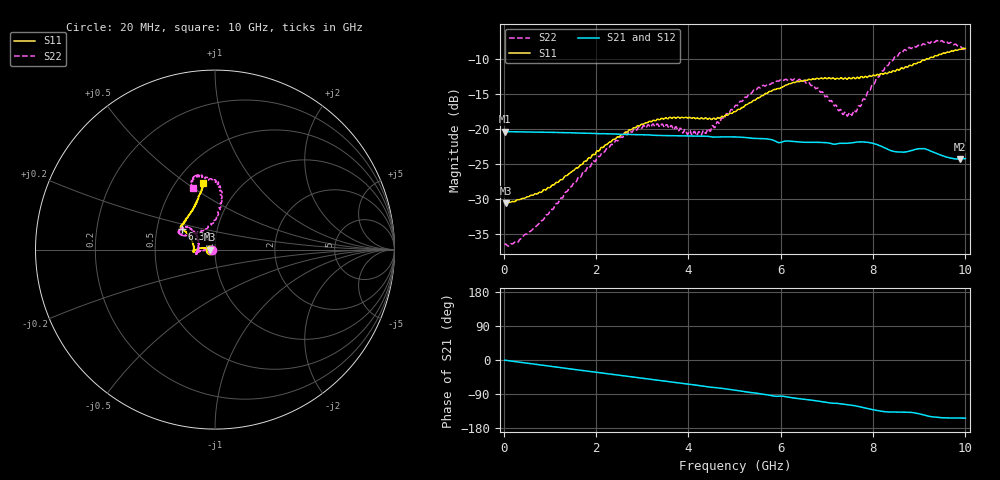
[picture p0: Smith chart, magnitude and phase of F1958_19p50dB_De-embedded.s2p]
! Integrated Device Technology
! Corporate Headquarters
! 6024 Silver Creek Valley Road
! San Jose, CA 95138  USA
! Phone:  1-408-284-8200
! Toll Free:  1-800-223-1366
! Webpage:  http://www.idt.com/
! Timing and RF Division
! 515 Groton Road, Suite 102
! Westford, MA 01886-6024
! Device:  F1958
! Description: 7-bit 0.25 dB Digital Step Attenuator
! Frequency:  0.001 -  6.000 GHz
! Package:  4x4 mm Thin QFN Plastic Package: 24 pin
! Ports:  2 RF, 12 DC
!  Pin  1  = D0
!  Pin  2  = VDD
!  Pin  3  = VMODE
!  Pin  4  = GND
!  Pin  5  = RF1  =  Port 1
!  Pin  6  = GND
!  Pin  7  = GND
!  Pin  8  = GND
!  Pin  9  = GND
!  Pin 10  = GND
!  Pin 11  = GND
!  Pin 12  = GND
!  Pin 13  = GND
!  Pin 14  = RF2  =  Port 2
!  Pin 15  = GND
!  Pin 16  = LE
!  Pin 17  = CLK
!  Pin 18  = DATA
!  Pin 19  = D6
!  Pin 20  = D5
!  Pin 21  = D4
!  Pin 22  = D3
!  Pin 23  = D2
!  Pin 24  = D1
! State:  78
! Atten State:  19.50 dB
! Voltage:  +3.30 Volts
! Current:  0.258 mA
! Data:  The device was measured on a F1958 evaluation board which has
!  individual transmission lines to the RF pins.  Data was collected
!  using a calibrated network analyzer.  The evaluation board was
!  de-embedded using Automatic Fixture Removal (AFR).
!  The reference plane is the edge of the package pin.
! Misc:
!  Action Tracker AT0419
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# GHz S dB R 50
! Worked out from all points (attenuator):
!   500 points, 20 MHz to 10 GHz, reference 50 ohm
!   highest |S21| = -20.38 dB at 20 MHz (marker M1); lowest = -24.3 dB at 9.88 GHz (marker M2)
!   lowest |S11| = -30.6 dB at 40 MHz (marker M3), VSWR 1.06, Z = 47.1 - j0.0432 ohm
!   |S11| at or under -10 dB: start of sweep to 9.159 GHz; 9.177217 GHz to 9.202731 GHz (25.51 MHz wide, 0.278 % of centre)
!   |S22| runs from -36.7 to -7.4 dB; largest |S21 - S12| = 0.00038
!   S11 on the Smith chart (normalised r, x): 20 MHz: 0.94, -0.00; 6.36 GHz: 0.67, +0.16; 10 GHz: 0.67, +0.58
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0.02  -30.54 -178.8  -20.38 -0.4  -20.38 -0.4  -36.53 -176.9
0.04  -30.58 -179.1  -20.38 -0.7  -20.38 -0.7  -36.41 -175.4
0.32  -30.09 175.2  -20.41 -5.4  -20.41 -5.3  -36.05 -179.0
0.72  -29.28 172.7  -20.45 -11.8  -20.44 -11.8  -33.78 -176.0
1.7  -25.06 171.4  -20.60 -27.5  -20.59 -27.5  -26.39 -177.4
2.6  -20.70 177.4  -20.76 -41.8  -20.74 -41.8  -20.96 -174.0
2.92  -19.55 -178.7  -20.81 -46.9  -20.79 -47.0  -19.73 -170.9
3.36  -18.68 -175.1  -20.93 -53.9  -20.92 -54.0  -19.56 -166.5
4.3  -18.45 -179.0  -21.03 -68.5  -21.04 -68.6  -20.58 164.7
4.64  -18.35 172.4  -21.14 -73.6  -21.15 -73.6  -19.00 151.8
5.02  -17.53 161.3  -21.13 -79.9  -21.14 -79.9  -16.62 140.3
5.58  -15.26 150.9  -21.38 -89.4  -21.39 -89.4  -14.04 140.3
6.36  -13.23 148.4  -21.83 -101.5  -21.85 -101.4  -13.14 153.8
6.68  -12.89 146.9  -21.90 -106.2  -21.91 -106.1  -13.79 154.9
7.32  -12.72 141.8  -22.06 -116.1  -22.06 -116.1  -17.53 134.4
7.5  -12.73 138.7  -22.01 -118.9  -22.01 -118.8  -17.67 116.2
7.68  -12.69 135.8  -21.85 -122.5  -21.85 -122.5  -16.72 98.5
8.34  -11.90 119.7  -22.96 -137.2  -22.96 -137.3  -10.80 82.5
8.68  -11.26 112.9  -23.30 -137.6  -23.28 -137.4  -8.68 86.9
9.26  -9.75 105.2  -23.18 -149.4  -23.19 -149.6  -7.56 99.8
9.88  -8.62 100.6  -24.29 -153.0  -24.32 -153.1  -8.22 109.2
10  -8.52 100.2  -24.21 -153.5  -24.22 -153.4  -8.77 110.0
